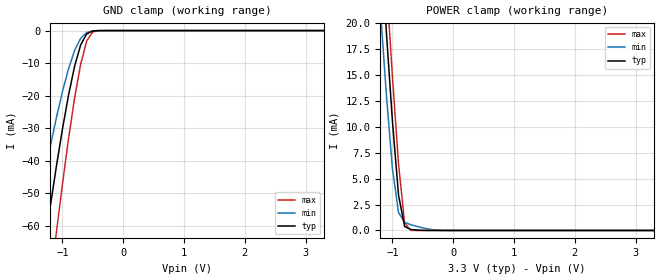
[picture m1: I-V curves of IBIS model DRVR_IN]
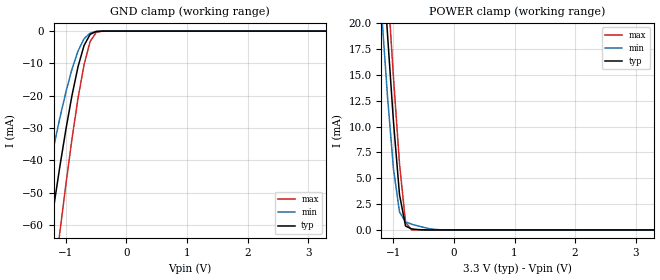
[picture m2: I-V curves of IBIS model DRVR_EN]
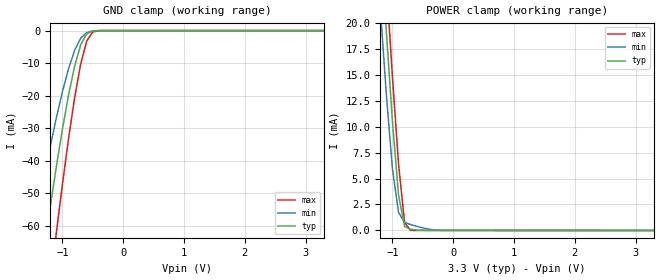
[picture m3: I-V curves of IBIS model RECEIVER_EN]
|   Texas Instruments Incorporated
|   High Speed Interface Products
|   IBIS Model for SN65MLVD204BRUM
|   16PIN RUM Package
[IBIS Ver]   4.2
[Comment char]   |_char
[File name]   sn65mlvd204brum.ibs
[File Rev]   1.2
[Date]   14Oct20
[Source]   File originated at Texas Instruments Incorporated.
   Data Transmission Products Group. All data based on
   Simulation Measurements.
[Notes]
   Revision 1.0
   - 30 Oct 2019
   - initial release
   Revision 1.1
   - 3 Sept 2020
   - Fixed typo in voltage range for DRIVE_OUT model
   Revision 1.2
   - 14 Oct 2020
   - Updated DRIVE_OUT model
[Disclaimer]
(C) Copyright Texas Instruments Incorporated 2020
   All rights reserved
  Texas Instruments Incorporated hereby grants the user of this IBIS
model a non-exclusive, nontransferable license to use this IBIS model
under the following terms.  Before using this IBIS model, the user
should read this license.  If the user does not accept these terms,
the IBIS model should be returned to Texas Instruments within 30 days.
  The user is granted this license only to use the IBIS model and
is not granted rights to sell, load, rent, lease or license the IBIS
model in whole or in part, or in modified form to anyone other than
user.  User may modify the IBIS model to suit its specific applications
but rights to derivative works and such modifications shall belong to
Texas Instruments.
  This IBIS model is provided on an "AS IS" basis and Texas Instruments
makes absolutely no warranty with respect to the information contained
herein.  TEXAS INSTRUMENTS DISCLAIMS AND CUSTOMER WAIVES ALL WARRANTIES,
EXPRESS OR IMPLIED, INCLUDING WARRANTIES OF MERCHANTABILITY OR FITNESS
FOR A PARTICULAR PURPOSE. The entire risk as to quality and performance
is with the Customer. ACCORDINGLY, IN NO EVENT SHALL THE COMPANY BE LIABLE
FOR ANY DAMAGES, WHETHER IN CONTRACT OR TORT,INCLUDING ANY LOST PROFITS
OR OTHER INCIDENTAL, CONSEQUENTIAL, EXEMPLARY, OR PUNITIVE DAMAGES ARISING
OUT OF THE USE OR APPLICATION OF THE IBIS model provided in this package.
Further, Texas Instruments reserves the right to discontinue or make changes
without notice to any product herein to improve reliability, function, or
design. Texas Instruments does not convey any license under patent rights
or any other intellectual property rights, including those of third parties.
Contact Texas Instruments at ATTN:DATA TRANSMISSIONS
[Copyright]   Copyright 2020, Texas Instruments, All Rights Reserved
[Component]   SN65MLVD204BRUM
[Manufacturer]  Texas Instruments Incorporated
[Package]
R_pkg 0.0777 0.042 0.109
L_pkg 8.16e-10 0.466e-9 1.115e-9
C_pkg 2.04e-13 0.172e-12 0.250e-12
[Pin]   signal_name   model_name   R_pin   L_pin   C_pin
1 R RECEIVER_OUT   0.108 1.093e-9 0.182e-12
2 RE_Z RECEIVER_EN   0.091 0.965e-9 0.184e-12
3 DE DRVR_EN   0.096 1.018e-9 0.188e-12
4 D DRVR_IN   0.109 1.115e-9 0.183e-12
5 GND GND   0.046 0.504e-9 0.222e-12
6 GND GND   0.042 0.466e-9 0.248e-12
10 A REC_IN_DRV_OUT   0.047 0.517e-9 0.235e-12
11 B REC_IN_DRV_OUT   0.048 0.535e-9 0.250e-12
13 VCC POWER   0.098 1.002e-9 0.172e-12
14 VCC POWER   0.091 0.944e-9 0.180e-12
[Diff_pin]   inv_pin   vdiff   tdelay_typ   tdelay_min   tdelay_max
10 11 0.15 0 0 0
[Model Selector] REC_IN_DRV_OUT
RECEIVER_IN   Differential receiver
DRIVER_OUT   Differential Driver
| Models and submodels in the file (6): DRVR_IN (Input), DRVR_EN (Input), RECEIVER_EN (Input), RECEIVER_IN (Input), DRIVER_OUT (3-state), RECEIVER_OUT (3-state)
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[Model]   DRVR_IN
Model_type   Input
Vinh=2.0
Vinl=0.8
|   typ min max
C_comp 1.58329e-12   1.57998e-12  1.60109e-12
[Temperature Range] 27.0 125.0 -40.0
[Voltage range]	 3.3 3.0 3.6
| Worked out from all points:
|   GND clamp passes 1 mA (typ) near -0.60 V on its own axis
|   POWER clamp passes 1 mA (typ) near -0.82 V on its own axis
[GND_clamp]
|   Voltage   I(typ)   I(min)   I(max)
-3.3V     -24.21A    -7.561A    -36.71A
-1.5V     -93.85mA   -65.37mA   -125.2mA
-1.4V     -80.26mA   -55.02mA   -109.1mA
-1.3V     -66.98mA   -45.09mA   -93.21mA
-1.2V     -54.12mA   -35.66mA   -77.5mA
-1.1V     -41.84mA   -26.85mA   -62.14mA
-900mV    -19.91mA   -11.77mA   -33.32mA
-800mV    -11mA      -6.118mA   -20.73mA
-700mV    -4.41mA    -2.358mA   -10.34mA
-600mV    -1.012mA   -605.6uA   -3.191mA
-400mV    -8.408uA   -10.91uA   -23.08uA
3.3V      1.65uA     1.55uA     2.007uA
[Power_clamp]
| Note that the[POWER_clamp]voltage table is referenced to Vcc
| and is calculated using Vtable=Vcc - Vmeasured.
|   Voltage   I(typ)   I(min)   I(max)
-1.898V   96.17mA    87.54mA    102mA
-1.199V   28.21mA    21.4mA     33.34mA
-1.099V   19.08mA    13.05mA    23.92mA
-999.7mV  10.51mA    5.932mA    14.81mA
-899.9mV  3.424mA    1.747mA    6.432mA
-800mV    381.6uA    782.6uA    746.8uA
-700mV    101.9uA    560uA      10.32uA
-400mV    2.586uA    124.5uA    2.251uA
-200mV    1.751uA    11.65uA    2.129uA
3.3V      -11.7pA    -194pA     -7.455pA
[Model]   DRVR_EN
Model_type   Input
Vinh=2.0
Vinl=0.8
|		 typ	 min	 max
C_comp 1.18741e-12  1.18345e-12		1.20433e-12
[Temperature Range]		 27.0	 125.0	 -40.0
[Voltage range]		 3.3	 3.0	 3.6
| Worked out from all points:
|   GND clamp passes 1 mA (typ) near -0.60 V on its own axis
|   POWER clamp passes 1 mA (typ) near -0.82 V on its own axis
[GND_clamp]
|   Voltage   I(typ)   I(min)   I(max)
-3.3V     -24.21A    -7.561A    -36.71A
-1.5V     -93.85mA   -65.37mA   -125.2mA
-1.4V     -80.26mA   -55.02mA   -109.1mA
-1.3V     -66.98mA   -45.09mA   -93.21mA
-1.2V     -54.12mA   -35.66mA   -77.5mA
-1.1V     -41.84mA   -26.85mA   -62.14mA
-900mV    -19.91mA   -11.77mA   -33.32mA
-800mV    -11mA      -6.118mA   -20.73mA
-700mV    -4.41mA    -2.358mA   -10.34mA
-600mV    -1.012mA   -605.6uA   -3.191mA
-400mV    -8.408uA   -10.91uA   -23.08uA
3.3V      1.65uA     1.55uA     2.007uA
[Power_clamp]
| Note that the[POWER_clamp]voltage table is referenced to Vcc
| and is calculated using Vtable=Vcc - Vmeasured.
|   Voltage   I(typ)   I(min)   I(max)
-1.898V   96.17mA    87.54mA    102mA
-1.199V   28.21mA    21.4mA     33.34mA
-1.099V   19.08mA    13.05mA    23.92mA
-999.7mV  10.51mA    5.932mA    14.81mA
-899.9mV  3.424mA    1.747mA    6.432mA
-800mV    381.6uA    782.6uA    746.8uA
-700mV    101.9uA    560uA      10.32uA
-400mV    2.586uA    124.5uA    2.251uA
-200mV    1.751uA    11.65uA    2.129uA
3.3V      -11.7pA    -194pA     -7.455pA
[Model]   RECEIVER_EN
Model_type   Input
Vinh=2.0
Vinl=0.8
|		 typ	 min	 max
C_comp 	1.18742e-12  1.18345e-12		1.20432e-12
[Temperature Range]		 27.0	 125.0	 -40.0
[Voltage range]		 3.3	 3.0	 3.6
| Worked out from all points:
|   GND clamp passes 1 mA (typ) near -0.60 V on its own axis
|   POWER clamp passes 1 mA (typ) near -0.82 V on its own axis
[GND_clamp]
|   Voltage   I(typ)   I(min)   I(max)
-3.3V     -24.21A    -7.561A    -36.71A
-1.5V     -93.85mA   -65.37mA   -125.2mA
-1.4V     -80.26mA   -55.02mA   -109.1mA
-1.3V     -66.98mA   -45.09mA   -93.21mA
-1.2V     -54.12mA   -35.66mA   -77.5mA
-1.1V     -41.84mA   -26.85mA   -62.14mA
-900mV    -19.91mA   -11.77mA   -33.33mA
-800mV    -11mA      -6.119mA   -20.74mA
-700mV    -4.412mA   -2.359mA   -10.34mA
-600mV    -1.014mA   -607uA     -3.194mA
-400mV    -11.88uA   -13.54uA   -27.58uA
3.3V      213pA      431.5nA    -364.8nA
[Power_clamp]
| Note that the[POWER_clamp]voltage table is referenced to Vcc
| and is calculated using Vtable=Vcc - Vmeasured.
|   Voltage   I(typ)   I(min)   I(max)
-1.898V   96.17mA    87.54mA    102mA
-1.199V   28.21mA    21.4mA     33.34mA
-1.099V   19.08mA    13.05mA    23.92mA
-999.7mV  10.51mA    5.932mA    14.81mA
-899.9mV  3.423mA    1.747mA    6.43mA
-800mV    380.9uA    782.6uA    745.1uA
-700mV    101.1uA    559.9uA    8.389uA
-400mV    1.15uA     124uA      121.7nA
-200mV    201.8nA    10.71uA    -121.5nA
3.3V      -3.298uA   -2.491uA   -4.378uA
